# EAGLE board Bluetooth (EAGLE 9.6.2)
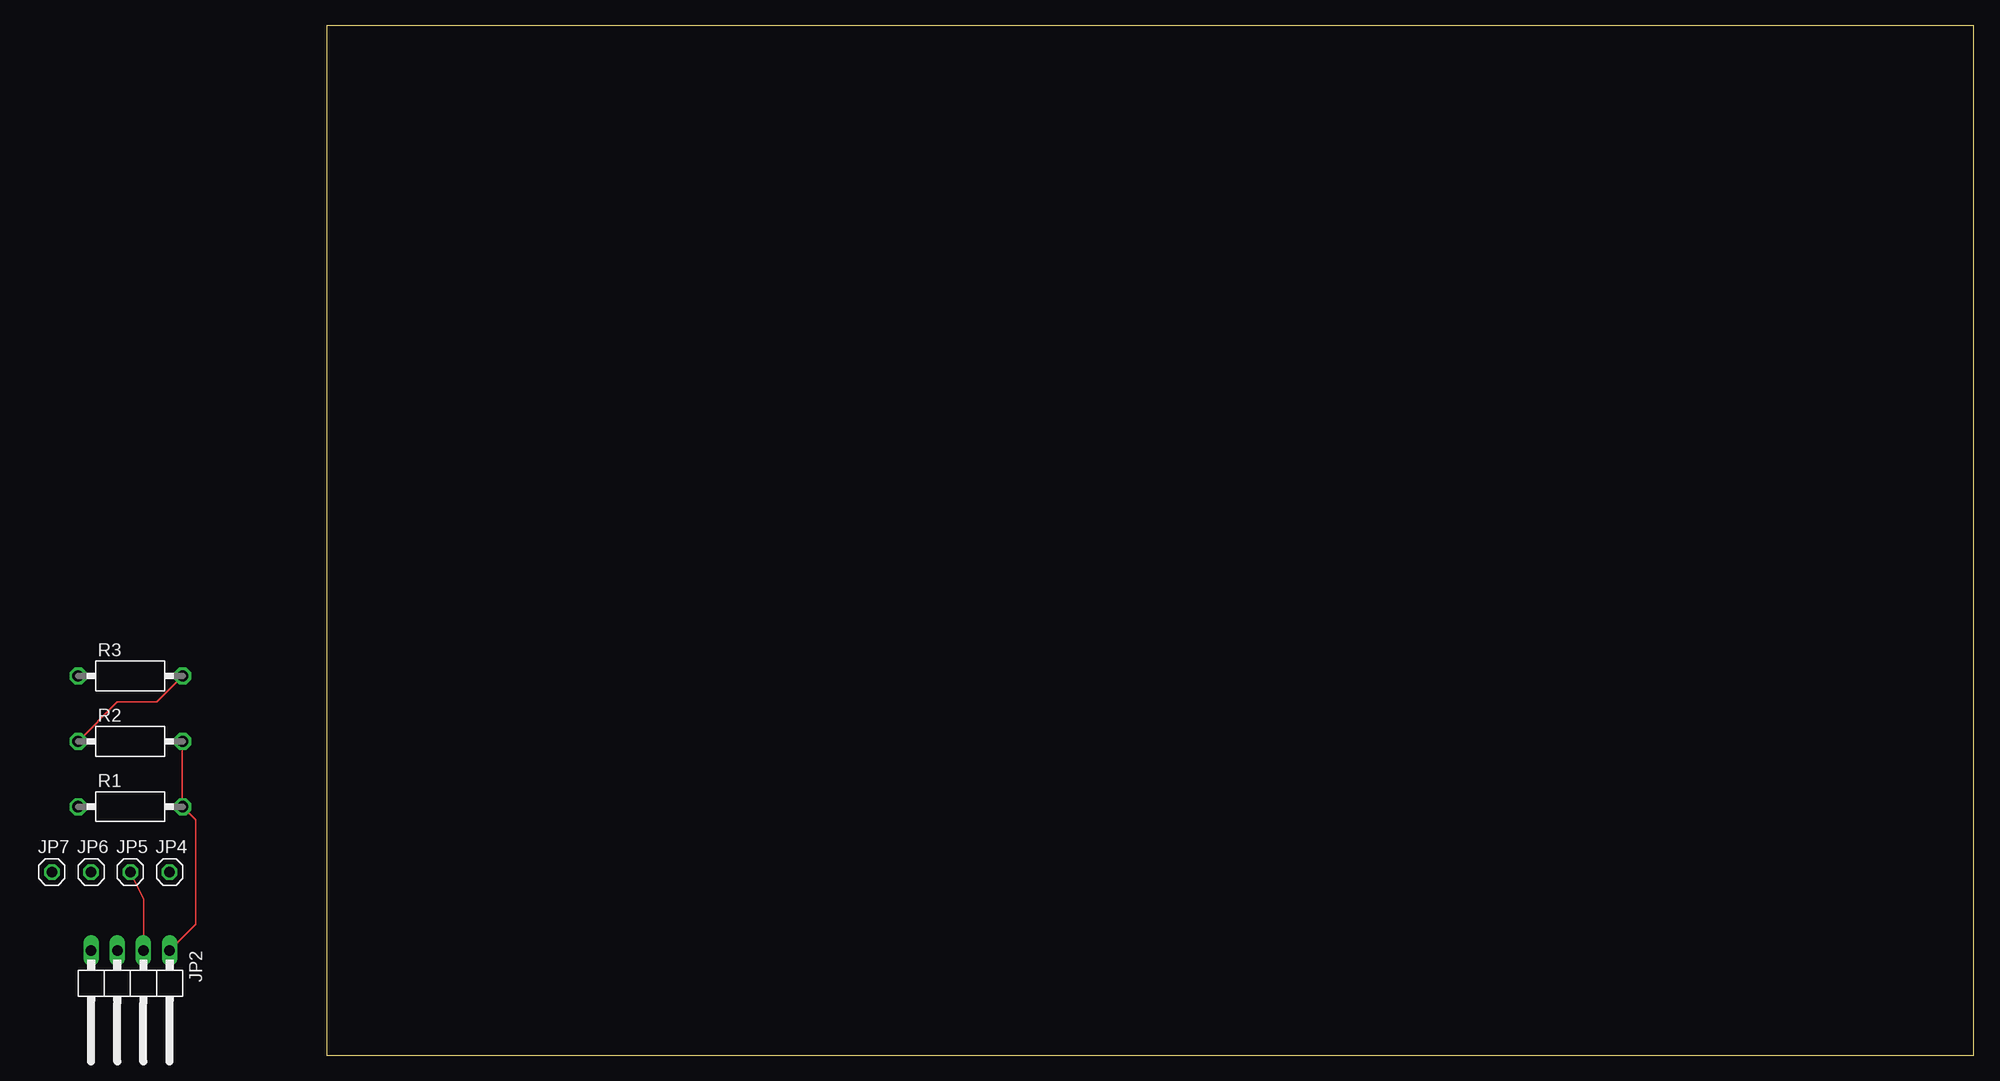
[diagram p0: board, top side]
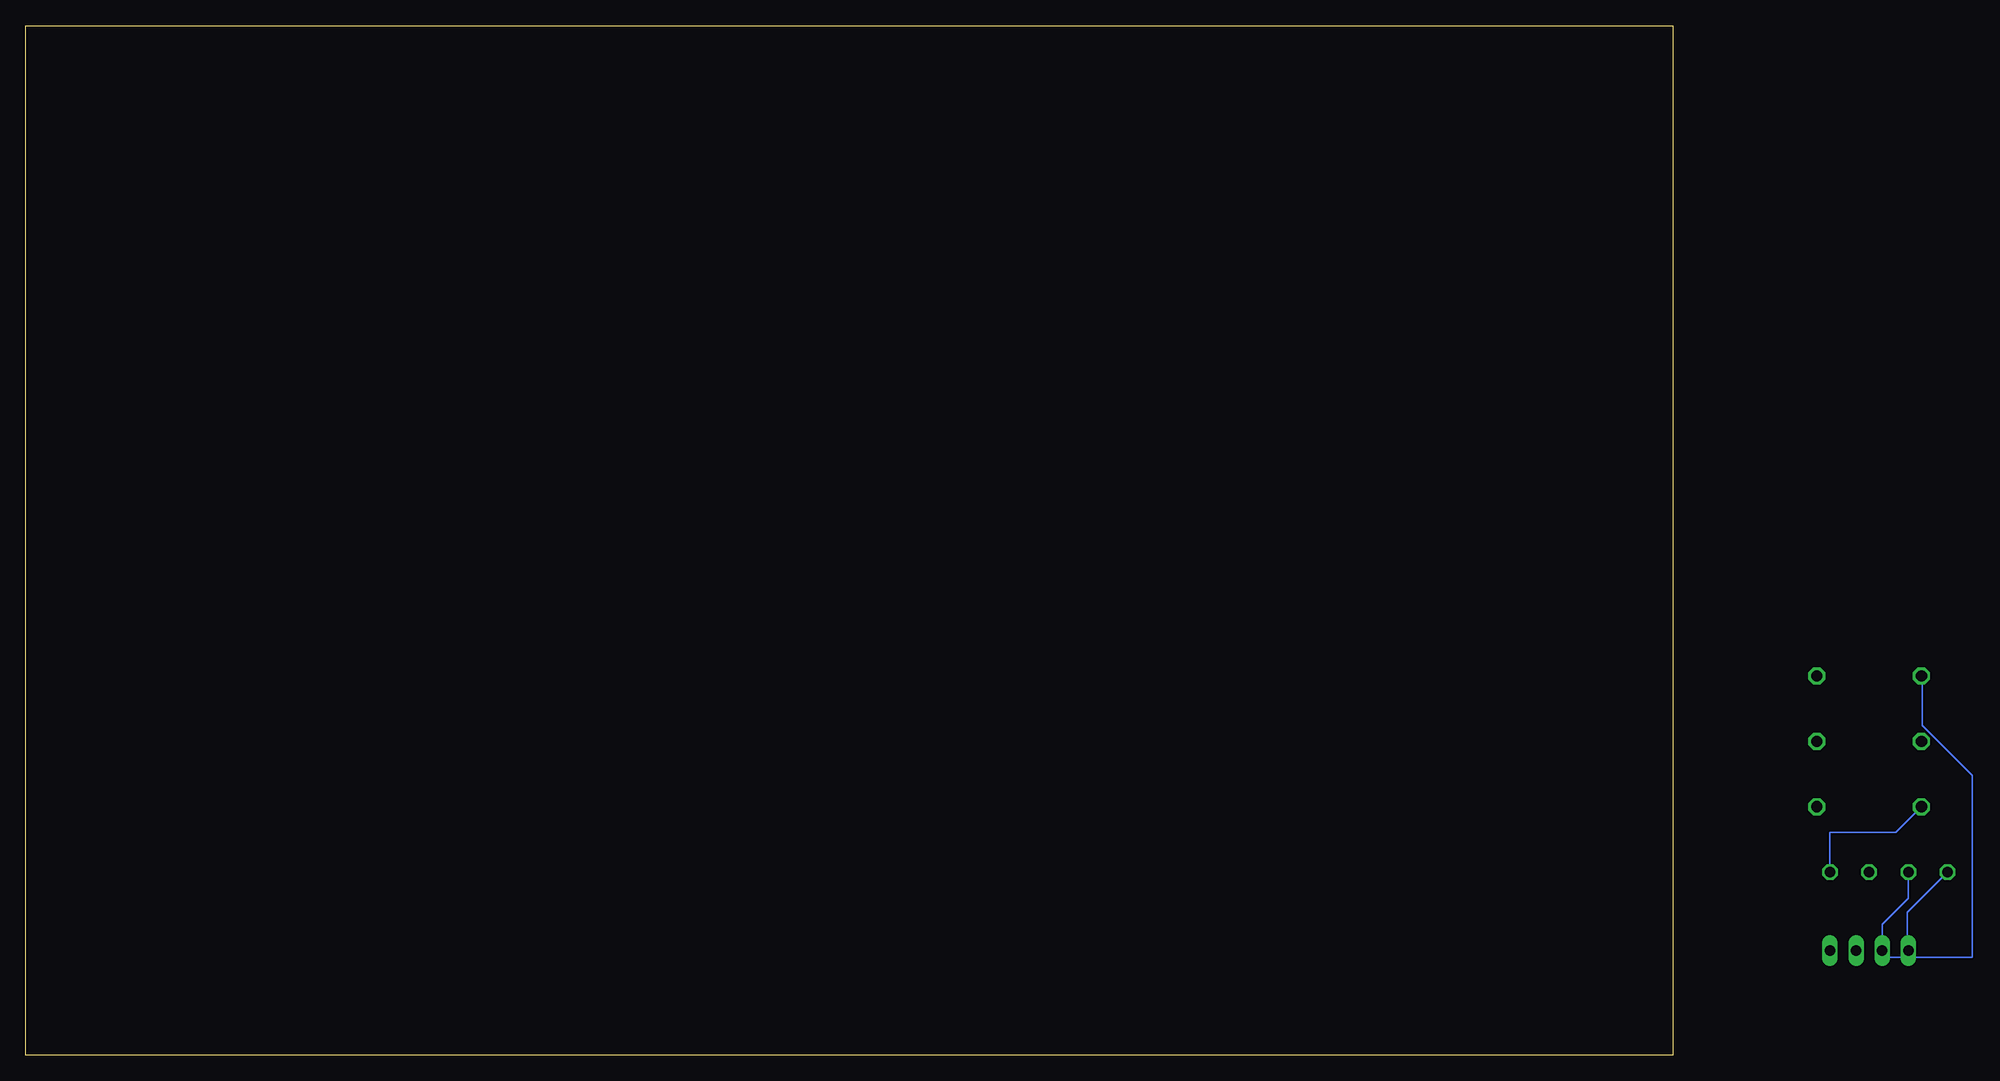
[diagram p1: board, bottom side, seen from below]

Size 160 x 100 mm. Coordinates in mm from the lower left corner, seen from the top.
Outline: 0,0 160,0 160,100 0,100 0,0
Copper layers (1*16): Top 0.035mm / dielectric 1.5mm / Bottom 0.035mm
Design rules "default": minimum track width 6mil, minimum drill 0.35mm, track to track 6mil, track to pad 6mil, pad to pad 6mil, via to via 6mil, smd to smd 6mil, copper to edge 40mil, drill to drill 6mil, minimum pad ring 10mil, minimum via ring 8mil, stop-mask expansion 4mil, vias tented up to drill 0mil, thermal gap 10mil

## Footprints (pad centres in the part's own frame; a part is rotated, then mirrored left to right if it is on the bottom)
1X04/90 = drill 1.016 long: 1 -3.81,-3.81; 2 -1.27,-3.81; 3 1.27,-3.81; 4 3.81,-3.81
1X01 = drill 1.016 octagon: 1 0,0
VMTA55 = drill 1.1 octagon: 1 -5.08,0; 2 5.08,0

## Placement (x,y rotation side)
JP2  [1X04/90]  -19.05,6.35 180 top  (outside the outline)
JP4  TX  [1X01]  -15.24,17.78 0 top  (outside the outline)
JP5  RX  [1X01]  -19.05,17.78 0 top  (outside the outline)
JP6  GND  [1X01]  -22.86,17.78 0 top  (outside the outline)
JP7  5 V  [1X01]  -26.67,17.78 0 top  (outside the outline)
R1  1K ohm  [VMTA55]  -19.05,24.13 0 top  (outside the outline)
R2  1K ohm  [VMTA55]  -19.05,30.48 0 top  (outside the outline)
R3  1K ohm  [VMTA55]  -19.05,36.83 0 top  (outside the outline)

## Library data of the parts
JP2 JP4-JP7 = pinhead
R1-R3 = rcl; SPICEPREFIX: R

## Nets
N$1: JP2.4 JP7.1
N$2: JP4.1 R1.1
N$3: JP2.2 JP5.1
N$4: JP2.1 R1.2 R2.2
N$5: JP2.3 JP6.1 R3.1
N$6: R2.1 R3.2

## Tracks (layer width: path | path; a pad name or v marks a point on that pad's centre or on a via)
N$1
  Bottom 0.152: JP2.4 -22.76,10.26 -22.76,13.87 JP7.1
N$2
  Bottom 0.152: R1.1 -21.64,21.64 -15.24,21.64 JP4.1
N$3
  Top 0.152: JP2.2 -17.73,10.21 -17.73,15.14 JP5.1
N$4
  Top 0.152: JP2.1 -12.7,12.7 -12.7,22.86 R1.2 -14.02,24.23 -14.02,30.48 R2.2
N$5
  Bottom 0.152: JP6.1 -22.86,15.24 -20.32,12.7 JP2.3 -20.32,9.5 -29.06,9.5 -29.06,27.18 -24.23,32 -24.23,36.73 R3.1
N$6
  Top 0.152: R2.1 -20.32,34.29 -16.51,34.29 R3.2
